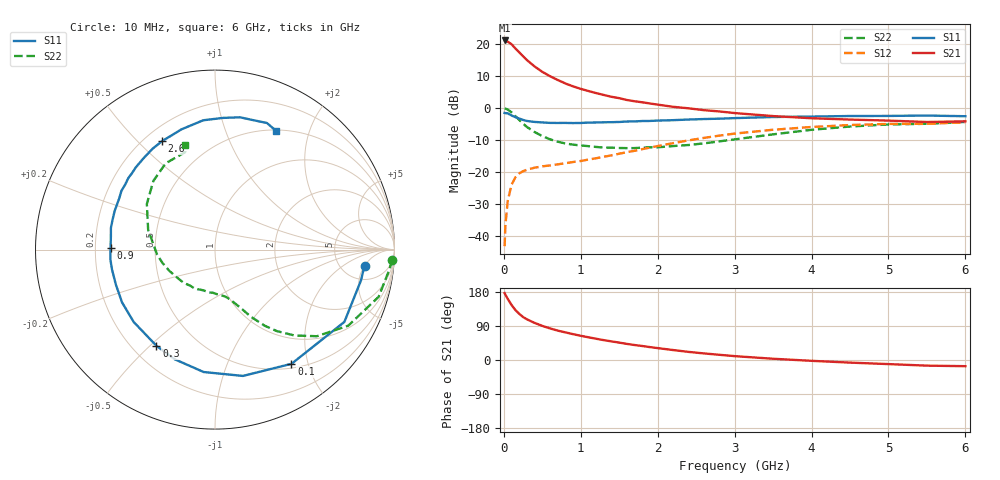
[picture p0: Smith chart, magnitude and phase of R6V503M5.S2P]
! SIEMENS Small Signal Semiconductors
! BFR193
! Si NPN RF Bipolar Junction Transistor in SOT23
! VCE = 0.5 V  IC = 3.5 mA
! Common Emitter S-Parameters:  May  1996
# GHz  S  MA  R  50
!  f  S11  S21  S12  S22
! GHz  MAG  ANG  MAG  ANG  MAG  ANG  MAG  ANG
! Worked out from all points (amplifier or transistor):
!   36 points, 10 MHz to 6 GHz, reference 50 ohm
!   highest |S21| = 21.1 dB at 10 MHz (marker M1)
!   |S21| within 3 dB of that: start of sweep to 170.9 MHz
!   unconditionally stable (mu >= 1): 932.4 MHz to 2.407 GHz; 5.242 GHz to end of sweep
!   at 250 MHz: K = 0.35, MSG = 17.9 dB, |S12| = -19.7 dB
!   at 1.4 GHz: K = 1.12, MAG = 7.0 dB, |S12| = -14.8 dB
!   at 6 GHz: K = 1.01, MAG = -0.3 dB, |S12| = -4.5 dB
!   S11 on the Smith chart (normalised r, x): 10 MHz: 8.32, -4.97; 100 MHz: 0.56, -1.73; 300 MHz: 0.30, -0.52; 900 MHz: 0.26, +0.01; 2.6 GHz: 0.27, +0.59; 6 GHz: 0.51, +1.51
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0.01  0.8377 -6.1  11.31 176.5  0.007 84.8  0.9886 -3.3
0.02  0.8313 -11.9  11.19 172.3  0.0146 83.5  0.9778 -6.6
0.05  0.8258 -29.2  10.84 161.5  0.0352 75.1  0.9489 -16.1
0.1  0.7659 -56.2  9.873 145.3  0.0636 62.3  0.8551 -29.7
0.15  0.7209 -77.5  8.487 131.8  0.0827 52.4  0.7447 -40.4
0.2  0.6849 -95.3  7.377 121.8  0.0956 46.0  0.6521 -47.2
0.25  0.6511 -110.1  6.407 113.4  0.1033 41.5  0.5701 -52.8
0.3  0.6276 -121.3  5.593 107.3  0.1089 38.8  0.5061 -56.9
0.4  0.6064 -138.3  4.445 97.9  0.1173 35.4  0.4218 -62.0
0.5  0.5956 -150.4  3.661 90.0  0.123 34.4  0.365 -65.5
0.6  0.5858 -160.4  3.134 83.4  0.1272 34.8  0.3246 -69.1
0.7  0.5845 -169.1  2.736 77.6  0.1321 35.8  0.2985 -72.1
0.9  0.5818 179.2  2.174 68.2  0.1437 38.2  0.2684 -77.5
1.1  0.5924 168.2  1.84 59.9  0.1569 41.2  0.254 -84.5
1.3  0.599 159.1  1.596 52.4  0.1738 44.0  0.241 -92.4
1.6  0.6156 147.9  1.332 42.5  0.2048 46.7  0.2366 -105.5
2.2  0.646 128.1  1.044 26.3  0.2829 46.1  0.2549 -133.8
2.6  0.6726 116.0  0.925 17.4  0.3415 42.2  0.2808 -155.1
3.5  0.7235 95.2  0.748 3.3  0.4577 28.2  0.3882 163.6
4.5  0.7502 79.3  0.66 -6.9  0.5423 12.0  0.5142 131.9
5.5  0.7624 67.7  0.605 -14.9  0.5674 -2.9  0.5673 107.2
6  0.7442 62.9  0.62 -16.3  0.5986 -7.3  0.6061 105.9
